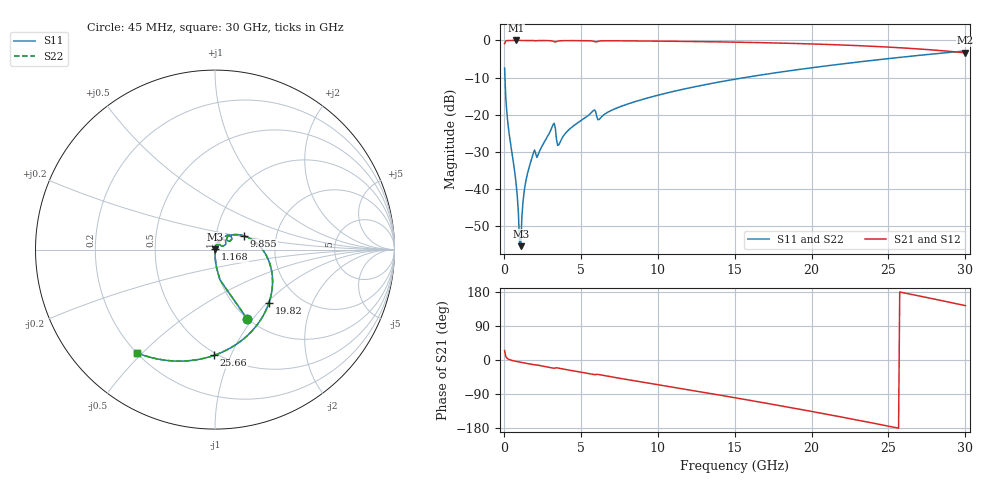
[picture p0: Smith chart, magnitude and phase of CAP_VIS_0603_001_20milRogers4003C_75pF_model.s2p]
! S-parameter model data by Modelithics Inc.  support@modelithics.com  813-866-6335  Tampa FL USA
! S-Parameter data specifications:
! Substrate: 20-mil Rogers 4003C, substrate thickness, H=0.508mm, Dielectric constant, Er=3.75
! PCB Mounting Pad Footprint: Pad width, PadW=0.90mm , Pad length, PadL=1.00mm , Pad gap, PadG (edge-to-edge)=1.00mm , Reference planes=3.0mm apart
! Created Wed Nov 18 13:30:11 2015
# hz S ma R 50
! 2 Port Network Data from SP1.SP block
! freq  magS11  angS11  magS21  angS21  magS12  angS12  magS22  angS22
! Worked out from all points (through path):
!   401 points, 45 MHz to 30 GHz, reference 50 ohm
!   highest |S21| = -0.01 dB at 793.9 MHz (marker M1); lowest = -3.3 dB at 30 GHz (marker M2)
!   group delay of S21, straight-line fit = 20 ps
!   lowest |S11| = -55.4 dB at 1.093 GHz (marker M3), VSWR 1.00, Z = 50.1 + j0.128 ohm
!   |S11| at or under -10 dB: 69.34 MHz to 15.65 GHz (15.58 GHz wide, 198 % of centre)
!   |S22| runs from -55.4 to -2.8 dB; largest |S21 - S12| = 0
!   S11 on the Smith chart (normalised r, x): 45 MHz: 1.00, -0.94; 1.168 GHz: 1.00, +0.01; 9.855 GHz: 1.37, +0.22; 19.82 GHz: 1.42, -1.03; 25.66 GHz: 0.48, -0.87; 30 GHz: 0.20, -0.48
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4.5e7  0.4246 -65.1  0.9052 24.9  0.9052 24.9  0.4246 -65.1
2.696625e8  0.07316 -86.9  0.9968 2.7  0.9968 2.7  0.07316 -86.9
7.93875e8  0.01176 -89.6  0.999 -3.7  0.999 -3.7  0.01176 -89.6
9.4365e8  0.004709 -83.7  0.999 -4.9  0.999 -4.9  0.004709 -83.7
1.093425e9  0.001707 48.4  0.9989 -6.0  0.9989 -6.0  0.001707 48.4
1.168312e9  0.004251 69.4  0.9989 -6.6  0.9989 -6.6  0.004251 69.4
1.318088e9  0.009315 75.4  0.9987 -7.7  0.9987 -7.7  0.009315 75.4
1.467862e9  0.01415 76.2  0.9985 -8.8  0.9985 -8.8  0.01415 76.2
1.917188e9  0.03053 69.9  0.9952 -12.2  0.9952 -12.2  0.03053 69.9
2.291625e9  0.03144 69.6  0.9959 -14.3  0.9959 -14.3  0.03144 69.6
3.190275e9  0.07342 52.6  0.977 -21.4  0.977 -21.4  0.07342 52.6
3.6396e9  0.04236 54.2  0.9889 -22.2  0.9889 -22.2  0.04236 54.2
5.062462e9  0.08496 55.3  0.9926 -32.4  0.9926 -32.4  0.08496 55.3
5.811338e9  0.1137 44.0  0.9775 -38.1  0.9775 -38.1  0.1137 44.0
9.855262e9  0.1797 25.0  0.9796 -64.0  0.9796 -64.0  0.1797 25.0
1.007992e10  0.1848 23.5  0.9786 -65.5  0.9786 -65.5  0.1848 23.5
1.50225e10  0.3009 -10.3  0.9484 -99.6  0.9484 -99.6  0.3009 -10.3
1.98153e10  0.4236 -44.9  0.8992 -134.3  0.8992 -134.3  0.4236 -44.9
2.003996e10  0.4296 -46.6  0.8963 -136.0  0.8963 -136.0  0.4296 -46.6
2.505742e10  0.5714 -85.6  0.8121 -175.1  0.8121 -175.1  0.5714 -85.6
2.565652e10  0.5893 -90.5  0.7991 -180.0  0.7991 -180.0  0.5893 -90.5
3e10  0.7211 -127.0  0.6817 143.5  0.6817 143.5  0.7211 -127.0
